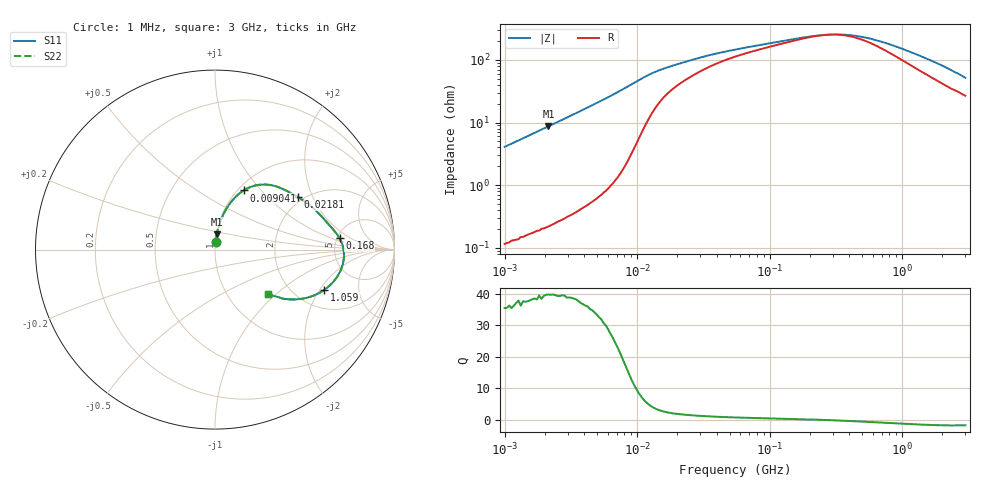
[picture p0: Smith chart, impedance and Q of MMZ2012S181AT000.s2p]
! S-parameter Generated by TDK Corporation
! Copyright(C) 2016 TDK Corporation.
! All Rights Reserved.
! TDK P/N: MMZ2012S181AT000 (Chip Beads)
! Property: |Z|=180¶ at 100MHz
! Size(LxWxT): 2x1.25x0.85mm, 0.079x0.049x0.033inches
! Model Type: s2p (Touchstone File Format Version 1.0)
! Frequency: DC=Yes Start=1MHz Stop=3000MHz 202points Log-sweep
! Note: This model was converted from impedance.
! Model Generated on May. 16, 2016
! Hash(MD5):
! Port Assignments:
!  1 ---@@@--- 2
! Applicable Conditions:
!  Temperature = 25 degC
!  DC Bias Current = 0 A
!  Small Signal Operation
! Terms and conditions regarding TDK Simulation Models
! (1)This simulation model is being provided solely for informational purposes. Please refer to the specifications of the products in terms of detailed characteristics of such products.
! (2)In no event shall TDK Corporation of any of its subsidiaries be liable for any loss or damage arising, directly or indirectly,
!  From any information contained in this simulation model, including, but not limited to loss or damages arising from any inaccuracies, omissions or errors in connection with such information.
! (3)Any and all copyrights on this simulation model are owned by TDK Corporation.
!  Duplication or redistribution of this simulation model without prior written permission from TDK Corporation is prohibited.
! (4)This simulation model is subject to any modification or change without any prior notice.
! (5)Neither TDK Corporation nor any of its subsidiaries shall make any warranty, express or implied,
!  Including but not limited to the correctness, implied warranties of merchantability and fitness for a particular purpose with respect to this simulation models.
! (6)The use of this simulation model shall be deemed to have consented to the terms and conditions hereof.
# MHz S MA R 50
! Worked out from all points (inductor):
!   201 points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, 1 MHz to 3 GHz, reference 50 ohm
!   read as one part in series: L = 647 nH near 1.041 MHz
!   highest Q = 39.7 at 2.14 MHz (marker M1), where L = 646 nH
!   self-resonance near 276.7 MHz
!   S11 on the Smith chart (normalised r, x): 1 MHz: 1.00, +0.08; 9.041 MHz: 1.06, +0.81; 21.81 MHz: 1.88, +1.57; 168 MHz: 5.26, +1.30; 1.059 GHz: 2.84, -2.21; 3 GHz: 1.53, -0.88
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1  0.04067 86.1  0.998 -2.3  0.998 -2.3  0.04067 86.1
2.13957  0.08637 83.6  0.9941 -5.0  0.9941 -5.0  0.08637 83.6
3.900413  0.1568 79.4  0.9834 -9.0  0.9834 -9.0  0.1568 79.4
6.305767  0.2546 73.2  0.9578 -14.7  0.9578 -14.7  0.2546 73.2
7.703107  0.3126 68.9  0.9342 -18.2  0.9342 -18.2  0.3126 68.9
9.040831  0.3665 64.1  0.9026 -21.4  0.9026 -21.4  0.3665 64.1
11.49534  0.4455 54.4  0.8245 -26.1  0.8245 -26.1  0.4455 54.4
14.61624  0.4974 44.1  0.7304 -28.3  0.7304 -28.3  0.4974 44.1
21.81181  0.5478 32.1  0.6099 -28.5  0.6099 -28.5  0.5478 32.1
33.87922  0.5938 23.0  0.509 -27.1  0.509 -27.1  0.5938 23.0
54.77226  0.6292 15.9  0.4311 -23.6  0.4311 -23.6  0.6292 15.9
168.0187  0.6966 5.2  0.3128 -11.7  0.3128 -11.7  0.6966 5.2
213.6344  0.708 2.8  0.2949 -6.8  0.2949 -6.8  0.708 2.8
306.2963  0.7184 -1.2  0.2822 3.0  0.2822 3.0  0.7184 -1.2
405.36  0.719 -4.7  0.2896 11.8  0.2896 11.8  0.719 -4.7
558.3748  0.7099 -9.3  0.3205 20.9  0.3205 20.9  0.7099 -9.3
800.5644  0.6837 -15.2  0.3843 27.7  0.3843 27.7  0.6837 -15.2
1059.487  0.6488 -20.3  0.4513 29.9  0.4513 29.9  0.6488 -20.3
1402.151  0.5988 -25.7  0.5288 29.4  0.5288 29.4  0.5988 -25.7
1855.641  0.5336 -31.3  0.6103 27.0  0.6103 27.0  0.5336 -31.3
2359.433  0.4637 -36.0  0.6817 23.6  0.6817 23.6  0.4637 -36.0
3000  0.385 -39.6  0.7451 19.2  0.7451 19.2  0.385 -39.6
